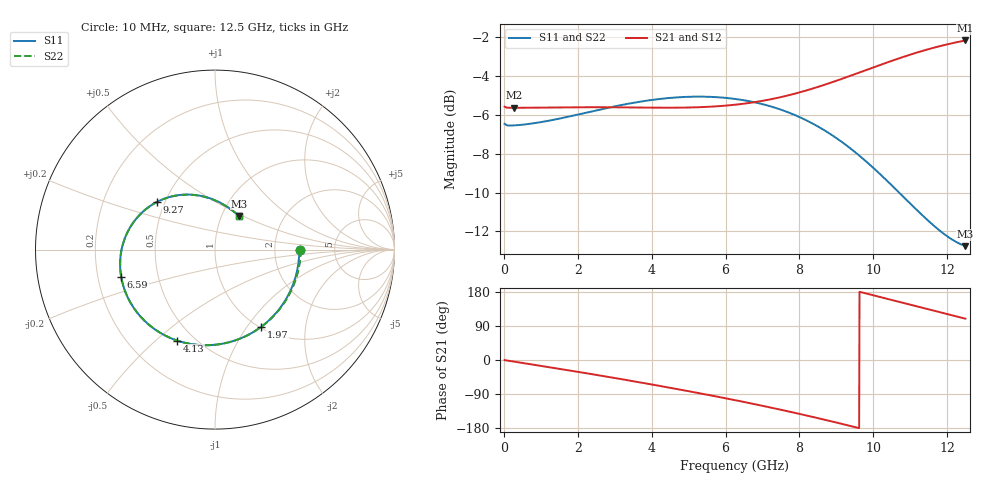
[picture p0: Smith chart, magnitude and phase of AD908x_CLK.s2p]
! Created Tue Jun 16 17:10:21 2020
# hz S ma R 50
! 2 Port Network Data from SP1.SP block
! freq  magS11  angS11  magS21  angS21  magS12  angS12  magS22  angS22
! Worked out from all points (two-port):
!   1250 points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, 10 MHz to 12.5 GHz, reference 50 ohm
!   highest |S21| = -2.18 dB at 12.5 GHz (marker M1); lowest = -5.6 dB at 270 MHz (marker M2)
!   |S21| within 3 dB of the highest: 7.293 GHz to end of sweep
!   lowest |S11| = -12.8 dB at 12.5 GHz (marker M3), VSWR 1.60, Z = 60.2 + j23.9 ohm
!   |S11| at or under -10 dB: 10.7 GHz to end of sweep
!   |S22| runs from -12.8 to -5.1 dB; largest |S21 - S12| = 0
!   S11 on the Smith chart (normalised r, x): 10 MHz: 2.81, -0.02; 1.97 GHz: 1.01, -1.17; 4.13 GHz: 0.40, -0.59; 6.59 GHz: 0.30, -0.13; 9.27 GHz: 0.45, +0.29; 12.5 GHz: 1.20, +0.48
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1e7  0.4752 -0.4  0.5259 -0.2  0.5259 -0.2  0.4751 -0.1
2.7e8  0.4707 -8.7  0.5223 -4.3  0.5223 -4.3  0.4778 -8.5
1.07e9  0.4813 -33.3  0.523 -16.7  0.523 -16.7  0.4844 -33.2
1.97e9  0.5013 -59.2  0.524 -30.8  0.524 -30.8  0.5018 -59.2
2.1e9  0.5045 -62.8  0.5241 -32.9  0.5241 -32.9  0.5048 -62.7
2.6e9  0.5171 -76.1  0.5242 -41.0  0.5242 -41.0  0.517 -76.0
3.1e9  0.5292 -88.7  0.5239 -49.3  0.5239 -49.3  0.529 -88.6
3.61e9  0.5402 -100.9  0.5233 -57.9  0.5233 -57.9  0.54 -100.8
4.13e9  0.5493 -112.7  0.5227 -66.9  0.5227 -66.9  0.549 -112.6
4.18e9  0.55 -113.9  0.5227 -67.8  0.5227 -67.8  0.5498 -113.7
5.27e9  0.5581 -137.1  0.5241 -87.3  0.5241 -87.3  0.5581 -137.0
6.26e9  0.5505 -157.2  0.532 -106.1  0.532 -106.1  0.5505 -157.1
6.59e9  0.5443 -163.8  0.5367 -112.6  0.5367 -112.6  0.5443 -163.7
7.45e9  0.5186 178.9  0.5552 -130.3  0.5552 -130.3  0.5184 179.0
8.34e9  0.4769 160.5  0.5846 -149.7  0.5846 -149.7  0.4767 160.7
9.27e9  0.4186 140.6  0.6259 -171.4  0.6259 -171.4  0.4186 140.8
9.86e9  0.3765 127.3  0.6559 174.3  0.6559 174.3  0.3765 127.6
1.042e10  0.3359 114.1  0.6855 160.5  0.6855 160.5  0.3357 114.4
1.09e10  0.303 102.1  0.7105 148.5  0.7105 148.5  0.3025 102.5
1.139e10  0.2732 89.0  0.7343 136.3  0.7343 136.3  0.2724 89.3
1.199e10  0.2447 71.3  0.76 121.5  0.76 121.5  0.244 71.5
1.25e10  0.2301 54.6  0.7785 109.1  0.7785 109.1  0.2299 54.7
